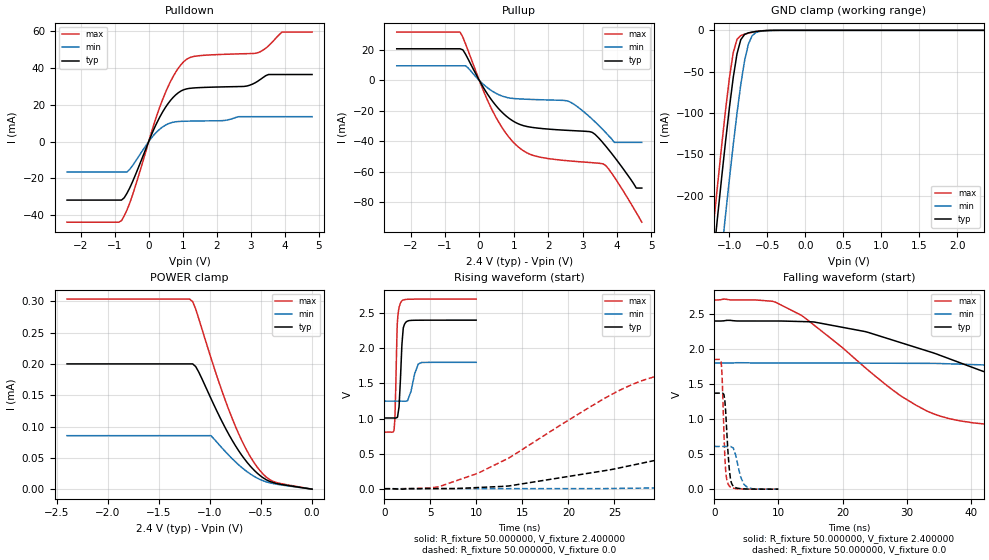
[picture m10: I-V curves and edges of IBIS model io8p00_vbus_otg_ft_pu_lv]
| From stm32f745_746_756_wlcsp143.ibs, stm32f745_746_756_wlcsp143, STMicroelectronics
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|   Model io8p00_vbus_otg_ft_pu_lv
[Model]  io8p00_vbus_otg_ft_pu_lv
Model_type I/O
Polarity   Non-Inverting
Enable   Active-Low
Vinl =   0.720000V
Vinh =   1.680000V
Vmeas =  1.200000V
Cref =   50.000000pF
Rref =   100.000000M
Vref =   0.0V
C_comp   3.193600pF   3.100000pF   3.332000pF
[Temperature Range]   25.000000   0.125000k   -40.000000
[Pullup Reference]   2.400000V   1.800000V   2.700000V
[Pulldown Reference]   0.0V   0.0V   0.0V
[POWER Clamp Reference]   2.400000V   1.800000V   2.700000V
[GND Clamp Reference]   0.0V   0.0V   0.0V
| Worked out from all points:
|   slope of the pulldown table from 0 to 0.36 V, typ, clamps not added: 25 ohm
|   slope of the pullup table from 0 to 0.36 V, typ, clamps not added: 27.7 ohm
|   GND clamp passes 1 mA (typ) near -0.61 V on its own axis
|   rising waveform, R_fixture 50.000000, V_fixture 2.400000: 20-80 % time 308ps typ, 629ps min, 212ps max; typ from 1.01 V to 2.4 V
|   rising waveform, R_fixture 50.000000, V_fixture 0.0: 20-80 % time 31ns typ, 72.9ns min, 14.4ns max; typ from 0.001 V to 1.37 V
|   falling waveform, R_fixture 50.000000, V_fixture 2.400000: 20-80 % time 29.3ns typ, 73.6ns min, 15.9ns max; typ from 2.4 V to 1.01 V
|   falling waveform, R_fixture 50.000000, V_fixture 0.0: 20-80 % time 574ps typ, 1.04ns min, 436ps max; typ from 1.37 V to 0.001 V
[Pulldown]
|Voltage   I(typ)   I(min)   I(max)
-2.4V     -31.69mA   -16.5mA    -43.66mA
-800mV    -31.69mA   -16.5mA    -42.82mA
-480mV    -21.96mA   -13.17mA   -29.19mA
80mV      3.63mA     1.966mA    5.014mA
480mV     18.16mA    8.738mA    26.02mA
800mV     25.38mA    10.72mA    37.77mA
1.12V     28.53mA    11.02mA    44.6mA
2.8V      29.84mA    13.46mA    47.53mA
3.2V      32.6mA     13.46mA    48.03mA
3.52V     36.28mA    13.46mA    51.75mA
3.92V     36.28mA    13.46mA    59.24mA
4.8V      36.28mA    13.46mA    59.24mA
[Pullup]
|Voltage   I(typ)   I(min)   I(max)
-2.4V     20.87mA    9.659mA    31.88mA
-560mV    20.87mA    9.659mA    31.88mA
-400mV    17.27mA    9.659mA    24.06mA
320mV     -11.75mA   -6.207mA   -17.08mA
960mV     -26.47mA   -11.82mA   -40.02mA
1.52V     -30.88mA   -12.51mA   -49.05mA
2.56V     -32.88mA   -13.49mA   -52.9mA
3.28V     -34.19mA   -25.52mA   -54.18mA
3.6V      -41.31mA   -32.62mA   -54.98mA
3.92V     -50.32mA   -40.8mA    -63.62mA
4.56V     -70.9mA    -40.8mA    -87.07mA
4.72V     -70.9mA    -40.8mA    -93.4mA
[GND_clamp]
|Voltage   I(typ)   I(min)   I(max)
-2.4V     -1.425A    -1.509A    -1.394A
-1.25V    -311.3mA   -401.9mA   -273.4mA
-1.2V     -265.5mA   -356.1mA   -227.3mA
-1.15V    -220.5mA   -310.9mA   -182mA
-1.1V     -176.4mA   -266.2mA   -138mA
-1.05V    -133.9mA   -222.5mA   -96.06mA
-950mV    -57.51mA   -139mA     -27.35mA
-900mV    -28.55mA   -100.5mA   -11.03mA
-850mV    -11.33mA   -65.67mA   -6.322mA
-750mV    -3.069mA   -16.69mA   -3.425mA
-600mV    -864.6uA   -1.294mA   -852.2uA
2.35V     0A         0A         0A
[POWER_clamp]
|Voltage   I(typ)   I(min)   I(max)
-2.4V     200uA      85.42uA    303.5uA
-1.2V     200uA      85.42uA    303.5uA
-1.17V    200uA      85.42uA    299.5uA
-1.14V    195.7uA    85.42uA    287.5uA
-990mV    144.6uA    85.42uA    209.3uA
-870mV    104.1uA    63.64uA    150.8uA
-780mV    77.28uA    48.22uA    111.8uA
-660mV    47.71uA    30.77uA    68.21uA
-570mV    30.64uA    20.64uA    42.8uA
-480mV    18.19uA    13.46uA    24.07uA
-390mV    10.91uA    9.255uA    13.01uA
0V        0A         0A         0A
[Ramp]
| variable   typ   min   max
dV/dt_r  0.82261/31.00235n   0.36231/74.73223n   1.11089/14.41169n
dV/dt_f  0.83664/29.33551n   0.32700/78.95536n   1.13654/15.86249n
R_load = 50.000000
[Rising Waveform]
R_fixture= 50.000000
V_fixture= 2.400000
V_fixture_min= 1.800000
V_fixture_max= 2.700000
|time   V(typ)   V(min)   V(max)
0s        1.007V     1.247V     805.7mV
1.041ns   1.007V     1.247V     839.2mV
1.141ns   1.007V     1.247V     1.04V
1.401ns   1.016V     1.247V     2.363V
1.582ns   1.163V     1.247V     2.574V
1.822ns   1.829V     1.247V     2.663V
2.042ns   2.288V     1.247V     2.687V
2.442ns   2.383V     1.249V     2.696V
3.684ns   2.399V     1.776V     2.699V
9.97ns    2.4V       1.8V       2.7V
[Rising Waveform]
R_fixture= 50.000000
V_fixture= 0.0
V_fixture_min= 0.0
V_fixture_max= 0.0
|time   V(typ)   V(min)   V(max)
0s        880.4uV    840.3uV    911.2uV
5.506ns   2.785mV    1.777mV    18.95mV
10.01ns   16.89mV    1.888mV    214.5mV
28.53ns   379.3mV    10.38mV    1.562V
36.04ns   601.7mV    22.76mV    1.736V
44.54ns   859.6mV    36.89mV    1.802V
61.06ns   1.192V     83.08mV    1.841V
82.08ns   1.323V     201.2mV    1.848V
144.1ns   1.368V     497.3mV    1.852V
249.2ns   1.371V     610.3mV    1.852V
[Falling Waveform]
R_fixture= 50.000000
V_fixture= 2.400000
V_fixture_min= 1.800000
V_fixture_max= 2.700000
|time   V(typ)   V(min)   V(max)
0s        2.4V       1.8V       2.7V
9.51ns    2.4V       1.8V       2.67V
14.01ns   2.391V     1.8V       2.452V
23.52ns   2.249V     1.799V     1.734V
31.53ns   2.02V      1.796V     1.193V
44.54ns   1.595V     1.766V     907.7mV
59.56ns   1.248V     1.714V     850.7mV
83.08ns   1.087V     1.581V     821.3mV
126.1ns   1.024V     1.378V     808.2mV
249.2ns   1.007V     1.247V     805.7mV
[Falling Waveform]
R_fixture= 50.000000
V_fixture= 0.0
V_fixture_min= 0.0
V_fixture_max= 0.0
|time   V(typ)   V(min)   V(max)
0s        1.371V     610.3mV    1.852V
1.061ns   1.371V     610.2mV    1.82V
1.241ns   1.371V     610.2mV    1.584V
1.682ns   1.237V     610mV      423.7mV
2.202ns   464mV      610.1mV    67.45mV
2.523ns   157.5mV    611.1mV    32.07mV
3.123ns   32.76mV    548.4mV    12.71mV
4.124ns   7.341mV    174.6mV    4.06mV
5.245ns   2.434mV    19.43mV    1.47mV
9.97ns    880.4uV    840.3uV    911.2uV
